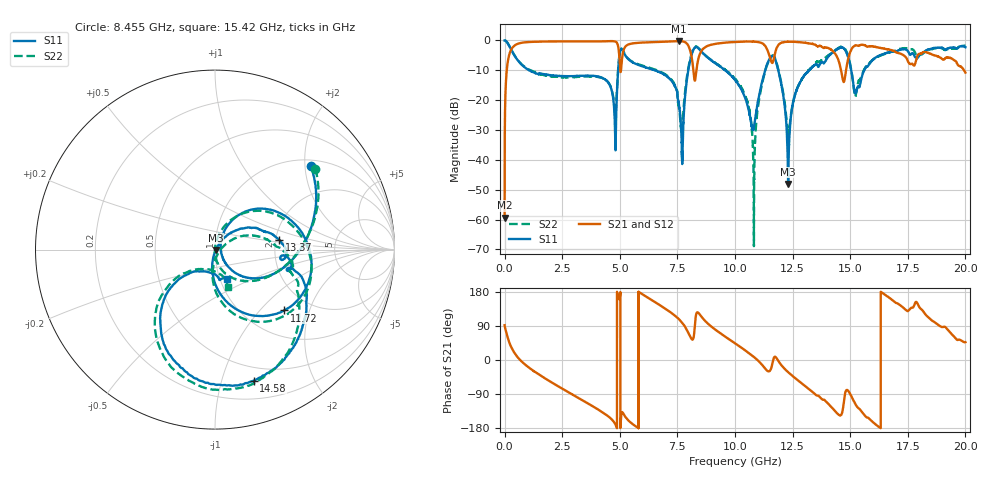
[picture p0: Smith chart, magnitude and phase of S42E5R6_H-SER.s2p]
! Created Wed Nov 25 21:47:24 2020
# khz S ma R 50
! 2 Port Network Data from SP1.SP block
! freq  magS11  angS11  magS21  angS21  magS12  angS12  magS22  angS22
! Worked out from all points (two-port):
!   20001 points, 300 kHz to 20 GHz, reference 50 ohm
!   highest |S21| = -0.21 dB at 7.577 GHz (marker M1); lowest = -59.3 dB at 300 kHz (marker M2)
!   |S21| within 3 dB of the highest: 276.7 MHz to 4.953 GHz (4.676 GHz wide, 179 % of centre); 5.166 GHz to 8.048 GHz (2.882 GHz wide, 43.6 % of centre)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
!   lowest |S11| = -48.0 dB at 12.31 GHz (marker M3), VSWR 1.01, Z = 50.3 - j0.205 ohm
!   |S11| at or under -10 dB: 1.07 GHz to 4.928 GHz (3.858 GHz wide, 129 % of centre); 6.521 GHz to 7.971 GHz (1.451 GHz wide, 20 % of centre); 9.573 GHz to 11.31 GHz (1.733 GHz wide, 16.6 % of centre)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
!   |S22| runs from -68.9 to 0.0 dB; largest |S21 - S12| = 0.02
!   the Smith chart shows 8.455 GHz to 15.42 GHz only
!   S11 on the Smith chart (normalised r, x): 8.455 GHz: 1.13, +2.14; 11.72 GHz: 1.49, -1.37; 13.37 GHz: 2.09, +0.26; 14.58 GHz: 0.37, -1.27; 15.42 GHz: 1.09, -0.36
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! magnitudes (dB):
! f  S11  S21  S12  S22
! 300 kHz  0.0  -59.3  -59.4  0.0
! 114.3 MHz  -0.7  -8.5  -8.5  -0.7
! 333.3 MHz  -3.8  -2.5  -2.5  -3.7
! 3.334 GHz  -11.9  -0.3  -0.3  -12.1
! 4.775 GHz  -25.8  -0.3  -0.3  -22.9
! 5.075 GHz  -2.8  -7.9  -7.9  -2.7
! 6.667 GHz  -10.4  -0.5  -0.5  -10.2
! 7.577 GHz  -22.0  -0.2  -0.2  -23.2
! 7.718 GHz  -39.5  -0.3  -0.3  -28.5
! 8.048 GHz  -6.9  -3.2  -3.2  -6.4
! 8.455 GHz  -3.0  -4.9  -5.0  -2.9
! 10 GHz  -13.2  -0.5  -0.5  -12.8
! 10.82 GHz  -29.2  -0.4  -0.4  -60.7
! 11.19 GHz  -13.3  -1.0  -1.0  -13.9
! 11.72 GHz  -5.8  -5.0  -5.0  -5.6
! 12.31 GHz  -48.0  -0.4  -0.4  -31.5
! 13.33 GHz  -9.1  -1.1  -1.1  -9.0
! 13.37 GHz  -8.8  -1.2  -1.2  -8.7
! 14.58 GHz  -2.4  -9.1  -9.1  -2.2
! 15.42 GHz  -15.1  -1.6  -1.5  -13.2
! 16.67 GHz  -4.0  -3.0  -3.2  -4.1
! 20 GHz  -2.3  -10.8  -10.7  -1.8
